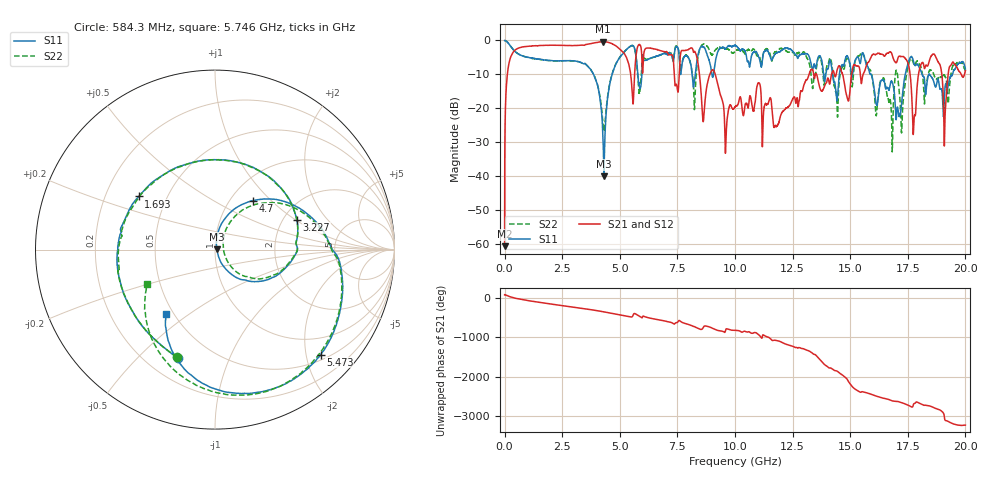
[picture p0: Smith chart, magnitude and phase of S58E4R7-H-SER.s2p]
!{S58E4R7}
!Johanson Technology Inc.
!www.johansontechnology.com
!Test Board Conditions:
!Substrate Type  RO4350B
!Substrate Thickness  60 mil
!Substrate Dk  3.66
!TL Type: GCPW
!TL Trace Width  115 mil
!TL Gap  52 mil
!Electrode orientation  Horizontal
!DUT TOPOLOGY	SERIES
!Mounting Pad LxW  55x428 mil
! Created Tue Apr 13 22:39:12 2021
# hz S ma R 50
! 2 Port Network Data from SP1.SP block
! freq  magS11  angS11  magS21  angS21  magS12  angS12  magS22  angS22
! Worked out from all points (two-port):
!   20001 points, 300 kHz to 20 GHz, reference 50 ohm
!   highest |S21| = -0.36 dB at 4.256 GHz (marker M1); lowest = -60.6 dB at 300 kHz (marker M2)
!   |S21| within 3 dB of the highest: 382.4 MHz to 5.121 GHz (4.738 GHz wide, 172 % of centre); 6.055 GHz to 7.055 GHz (1 GHz wide, 15.3 % of centre)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
!   lowest |S11| = -39.9 dB at 4.311 GHz (marker M3), VSWR 1.02, Z = 51 + j0.0788 ohm
!   |S11| at or under -10 dB: 3.861 GHz to 4.665 GHz (804.5 MHz wide, 18.9 % of centre); 15.91 GHz to 17.39 GHz (1.476 GHz wide, 8.87 % of centre); 18.44 GHz to 19.44 GHz (998.5 MHz wide, 5.27 % of centre)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
!   |S22| runs from -32.8 to 0.0 dB; largest |S21 - S12| = 0.011
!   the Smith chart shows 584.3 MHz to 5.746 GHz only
!   S11 on the Smith chart (normalised r, x): 584.3 MHz: 0.33, -0.66; 1.693 GHz: 0.35, +0.28; 3.227 GHz: 2.37, +1.02; 4.7 GHz: 1.27, +0.79; 5.473 GHz: 0.61, -2.29; 5.746 GHz: 0.46, -0.40
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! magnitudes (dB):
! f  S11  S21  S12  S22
! 300 kHz  0.0  -60.6  -60.7  0.0
! 143.3 MHz  -0.6  -8.6  -8.6  -0.7
! 584.3 MHz  -3.9  -2.3  -2.3  -3.9
! 1.693 GHz  -5.7  -1.5  -1.5  -5.8
! 3.227 GHz  -6.3  -1.4  -1.4  -6.3
! 3.334 GHz  -6.5  -1.4  -1.4  -6.5
! 4.256 GHz  -26.0  -0.4  -0.4  -23.5
! 4.311 GHz  -39.9  -0.4  -0.4  -26.5
! 4.7 GHz  -9.2  -1.1  -1.1  -9.2
! 5.473 GHz  -1.6  -10.1  -10.1  -1.7
! 5.746 GHz  -7.1  -2.6  -2.6  -7.6
! 6.667 GHz  -4.5  -2.8  -2.8  -4.5
! 10 GHz  -1.5  -19.6  -19.4  -3.3
! 11.78 GHz  -3.7  -25.3  -25.3  -3.4
! 13.33 GHz  -7.8  -8.4  -8.4  -12.4
! 15.51 GHz  -3.9  -11.7  -11.6  -3.4
! 16.67 GHz  -14.5  -3.7  -3.7  -17.8
! 17.47 GHz  -7.7  -6.1  -6.0  -8.8
! 17.77 GHz  -6.8  -23.1  -22.9  -7.3
! 18.57 GHz  -11.1  -4.2  -4.2  -9.0
! 19.11 GHz  -14.3  -24.0  -24.1  -10.5
! 20 GHz  -8.4  -8.9  -8.9  -8.9
